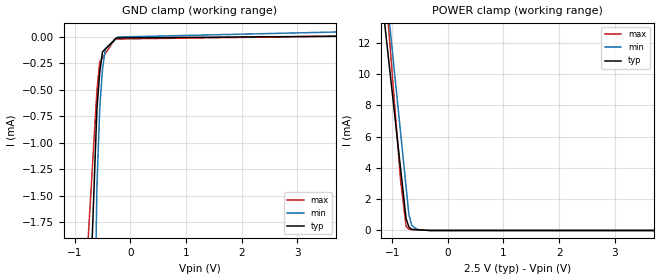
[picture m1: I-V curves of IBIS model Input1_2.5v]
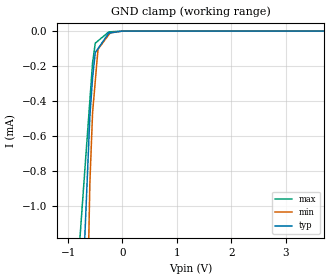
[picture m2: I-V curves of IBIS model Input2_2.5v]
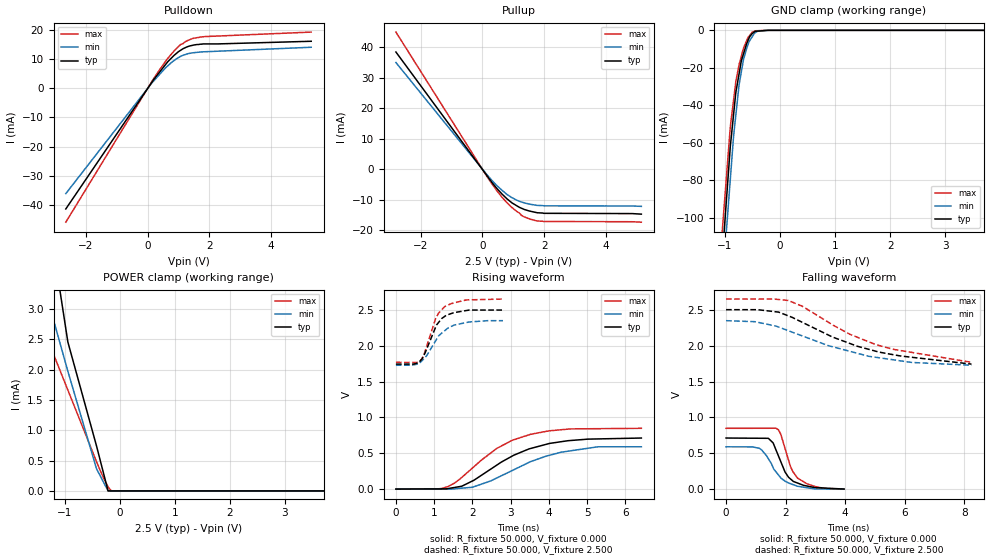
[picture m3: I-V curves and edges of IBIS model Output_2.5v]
[IBIS Ver]   3.2
[Comment Char] |_char
[File Name]   ads7886sbdckt.ibs
[File Rev]   3.0
[Source]
| This model file was created by Teraspeed Consulting Group LLC
| (http://www.teraspeed.com/).
[Date]   08-24-2006
[Notes]   Quality Check of this IBIS model: Model Passes IBIS Check
   Model parses into ICX IS. Simulation done with Hyperlynx.
   1. MIN TYP MAX information is based on Temprature and Voltage
   characteristics only.
[Disclaimer]
| This model is designed as an aid for customers of Texas Instruments.
| TI and its licensors and suppliers make no warranties, either expressed
| or implied, with respect to this  model, including the warranties of
| merchantability or fitness for a particular purpose.
| The model is provided solely on an "as is" basis. The entire risk as to
| its quality and performance is with the customer.
[Copyright]
| (C) Copyright 2008 Texas Instruments Incorporated. All rights reserved.
[Component] ads7886sbdckt
[Manufacturer] TI
[Package]
| variable   typ   min   max
R_pkg  1.00E-02 1.00E-02 1.00E-02
L_pkg  7.45E-09   3.43E-09 1.26E-08
C_pkg  2.00E-12   1.10E-12 3.17E-12
[Pin] signal_name  model_name  R_pin  L_pin C_pin
1   VDD  POWER   1.00E-02  1.26E-08  3.17E-12
2   GND  GND   1.00E-02  9.36E-09  3.13E-12
3   VIN  Input1   1.00E-02  6.47E-09  1.54E-12
4   SCLK Input2   1.00E-02  6.42E-09  1.54E-12
5   SDO  Output   1.00E-02  3.43E-09  1.10E-12
6   _CS  Input2   1.00E-02  6.42E-09  1.54E-12
[Model Selector] Input1
Input1_2.5v   2.5v analog input
Input1_3.3v   3.3v analog input
Input1_5v   5v analog input
[Model Selector] Input2
Input2_2.5v   2.5v cmos input
Input2_3.3v   3.3v cmos input
Input2_5v   5v cmos input
[Model Selector] Output
Output_2.5v   2.5v cmos output
Output_3.3v   3.3v cmos output
Output_5v   5v cmos output
| Models and submodels in the file (9): Input1_2.5v (Terminator), Input2_2.5v (Input), Output_2.5v (3-state), Input1_3.3v (Terminator), Input2_3.3v (Input), Output_3.3v (3-state), Input1_5v (Terminator), Input2_5v (Input), Output_5v (3-state)
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[Model] Input1_2.5v
Model_type Terminator
C_comp 1.513pF 1.513pF 1.513pF
| variable typ   min   max
[Voltage Range] 2.50000V 2.35000V 2.65000V
[POWER Clamp Reference] 2.50000V 2.35000V 2.65000V
[GND Clamp Reference] 0.00000V 0.00000V 0.00000V
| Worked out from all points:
|   POWER clamp passes 1 mA (typ) near -0.76 V on its own axis
[GND Clamp]
-2.5V     -28.03mA   -65.65mA   -17.39mA
-600mV    -679.7uA   -1.408mA   -508.4uA
-550mV    -338.1uA   -679.4uA   -237.9uA
-500mV    -141uA     -306.6uA   -198.4uA
-450mV    -114.9uA   -118.7uA   -159uA
-275mV    -23.6uA    -27.84uA   -20.92uA
-250mV    -10.55uA   -14.86uA   -20.75uA
-225mV    -10.45uA   -1.878uA   -20.58uA
5V        10.35uA    61.07uA    14.79uA
[POWER Clamp]
-2.5V     57.53mA    64.44mA    78.26mA
-950mV    7.245mA    9.833mA    7.794mA
-850mV    4.001mA    6.311mA    3.247mA
-750mV    757.4uA    2.788mA    268.8uA
-700mV    229.4uA    1.026mA    79.28uA
-650mV    66.25uA    332uA      69.95uA
-550mV    45.87uA    65.59uA    51.3uA
-325mV    0A         0A         9.327uA
5V        0A         0A         0A
[Model] Input2_2.5v
Model_type Input
Vinl = 400.000mV
Vinh = 4.60000V
C_comp 1.513pF 1.513pF 1.513pF
| variable typ   min   max
[Voltage Range] 2.50000V 2.35000V 2.65000V
[POWER Clamp Reference] 2.50000V 2.35000V 2.65000V
[GND Clamp Reference] 0.00000V 0.00000V 0.00000V
[GND Clamp]
-2.5V     -14.64mA   -31.06mA   -8.604mA
-600mV    -491.1uA   -875.5uA   -398.6uA
-550mV    -268.7uA   -469.1uA   -182.7uA
-500mV    -122.8uA   -286.4uA   -68.95uA
-450mV    -100.3uA   -103.7uA   -55.99uA
-250mV    -10.46uA   -20.52uA   -4.143uA
-225mV    -10.42uA   -10.12uA   -4.122uA
0V        0A         0A         0A
5V        0A         0A         0A
[POWER Clamp]
-2.5V     0A         0A         0A
5V        0A         0A         0A
[Model] Output_2.5v
Model_type 3-state
Vref=0.00000V
Rref=5.00000Mohms
Cref=50.0000pF
Vmeas=1.25000V
C_comp 1.513pF 1.513pF 1.513pF
| variable typ   min   max
[Voltage Range] 2.50000V 2.35000V 2.65000V
[POWER Clamp Reference] 2.50000V 2.35000V 2.65000V
[Pullup Reference] 2.50000V 2.35000V 2.65000V
[Pulldown Reference] 0.00000V 0.00000V 0.00000V
[GND Clamp Reference] 0.00000V 0.00000V 0.00000V
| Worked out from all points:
|   slope of the pulldown table from 0 to 0.375 V, typ, clamps not added: 68.6 ohm
|   slope of the pullup table from 0 to 0.375 V, typ, clamps not added: 73.8 ohm
|   GND clamp passes 1 mA (typ) near -0.47 V on its own axis
|   POWER clamp passes 1 mA (typ) near -0.50 V on its own axis
|   rising waveform, R_fixture 50.000, V_fixture 0.000: 20-80 % time 1.45ns typ, 1.52ns min, 1.3ns max; typ from 0.002 V to 0.713 V
|   falling waveform, R_fixture 50.000, V_fixture 0.000: 20-80 % time 506ps typ, 616ps min, 473ps max; typ from 0.713 V to 0.002 V
|   falling waveform, R_fixture 50.000, V_fixture 2.500: 20-80 % time 2.9ns typ, 2.81ns min, 2.82ns max; typ from 2.5 V to 1.74 V
|   rising waveform, R_fixture 50.000, V_fixture 2.500: 20-80 % time 391ps typ, 521ps min, 373ps max; typ from 1.74 V to 2.5 V
[GND Clamp]
-2.65V    -772.7mA   -757.1mA   -716.5mA
-2.35V    -650.9mA   -640.9mA   -602.5mA
-900mV    -62.01mA   -79.51mA   -51.55mA
-840mV    -44.75mA   -56.28mA   -37.07mA
-800mV    -33.24mA   -45.33mA   -27.42mA
-740mV    -23.07mA   -28.92mA   -18.2mA
-660mV    -12.51mA   -15.49mA   -9.444mA
-560mV    -4.16mA    -6.07mA    -3.126mA
-500mV    -1.63mA    -3.31mA    -923.7uA
-400mV    -420.1uA   -392.6uA   -189.9uA
-200mV    0A         0A         0A
5.3V      0A         0A         0A
[Pulldown]
-2.65V    -41.4mA    -36.14mA   -45.94mA
200mV     3.032mA    2.556mA    3.353mA
650mV     9.078mA    7.679mA    10.21mA
850mV     11.23mA    9.47mA     12.72mA
1.08V     13.12mA    11.01mA    15.09mA
1.15V     13.59mA    11.33mA    15.31mA
1.25V     14.1mA     11.69mA    16.14mA
1.44V     14.71mA    12.16mA    17.02mA
1.88V     15.23mA    12.55mA    17.76mA
5.3V      16.14mA    14.09mA    19.29mA
[Pullup]
-2.8V     38.44mA    35mA       44.98mA
150mV     -2.107mA   -1.8mA     -2.378mA
320mV     -4.444mA   -3.781mA   -4.906mA
640mV     -8.159mA   -6.919mA   -9.216mA
800mV     -9.715mA   -8.281mA   -10.99mA
960mV     -11.03mA   -9.319mA   -12.56mA
1.2V      -12.48mA   -10.5mA    -14.36mA
1.26V     -12.74mA   -10.71mA   -15.06mA
1.54V     -13.72mA   -11.45mA   -16.32mA
1.74V     -14.17mA   -11.79mA   -16.89mA
1.98V     -14.44mA   -11.98mA   -17.12mA
5.15V     -14.71mA   -12.16mA   -17.35mA
[POWER Clamp]
-2.8V     13.74mA    8.011mA    5.881mA
-2.2V     9.89mA     6.064mA    4.52mA
-940mV    2.455mA    1.974mA    1.663mA
-420mV    742.5uA    365.9uA    483.3uA
-325mV    406.6uA    200.4uA    278.2uA
-210mV    0A         0A         64.92uA
-150mV    0A         0A         0A
5.15V     0A         0A         0A
[Rising Waveform]
R_fixture = 50.000
V_fixture = 0.000
V_fixture_min = 0.000
V_fixture_max = 0.000
|  time   V(typ)   V(min)   V(max)
0s        2.411mV    1.619mV    866.7uV
1.04ns    4.754mV    1.94mV     2.795mV
1.36ns    8.978mV    2.039mV    36.54mV
1.72ns    41.32mV    14.68mV    163.4mV
2ns       114.5mV    27.29mV    294.7mV
2.64ns    336.6mV    157mV      569.1mV
3.52ns    567.2mV    384.1mV    764.8mV
4.32ns    661.7mV    515.5mV    828.5mV
5.28ns    700.7mV    590.9mV    843.4mV
6.42ns    713.2mV    590.9mV    848.5mV
[Falling Waveform]
R_fixture = 50.000
V_fixture = 0.000
V_fixture_min = 0.000
V_fixture_max = 0.000
|  time   V(typ)   V(min)   V(max)
0s        713.2mV    590.9mV    848.5mV
1.12ns    710.1mV    569.6mV    849.2mV
1.42ns    709.3mV    425.2mV    849.4mV
1.68ns    544.2mV    240.2mV    849.5mV
1.84ns    382.1mV    156.8mV    763.1mV
1.98ns    240.2mV    113.8mV    569.2mV
2.16ns    144.3mV    77.64mV    319.8mV
2.4ns     86.24mV    41.31mV    155.1mV
3.04ns    22.44mV    4.712mV    31.38mV
3.96ns    2.411mV    1.619mV    866.7uV
[Falling Waveform]
R_fixture = 50.000
V_fixture = 2.500
V_fixture_min = 2.350
V_fixture_max = 2.650
|  time   V(typ)   V(min)   V(max)
0s        2.501V     2.348V     2.649V
960ps     2.501V     2.334V     2.649V
1.76ns    2.468V     2.26V      2.643V
2.08ns    2.417V     2.21V      2.63V
2.56ns    2.325V     2.136V     2.549V
3.58ns    2.119V     1.984V     2.289V
4.16ns    2.03V      1.921V     2.158V
5.04ns    1.921V     1.837V     2.013V
6.24ns    1.838V     1.766V     1.906V
8.24ns    1.743V     1.727V     1.768V
[Rising Waveform]
R_fixture = 50.000
V_fixture = 2.500
V_fixture_min = 2.350
V_fixture_max = 2.650
|  time   V(typ)   V(min)   V(max)
0s        1.743V     1.727V     1.768V
460ps     1.743V     1.733V     1.766V
640ps     1.791V     1.768V     1.787V
720ps     1.854V     1.812V     1.852V
1.04ns    2.26V      2.068V     2.38V
1.12ns    2.326V     2.139V     2.457V
1.28ns    2.409V     2.21V      2.545V
1.52ns    2.46V      2.286V     2.595V
1.92ns    2.496V     2.33V      2.638V
2.8ns     2.496V     2.348V     2.649V
[Ramp]
| variable typ min max
dV/dt_r 426.666m/1.14425n 353.644m/1.32326n 509.557m/1.04296n
dV/dt_f 455.009m/2.53400n 372.615m/2.82000n 528.929m/2.25823n
R_load = 50.0000Ohms
